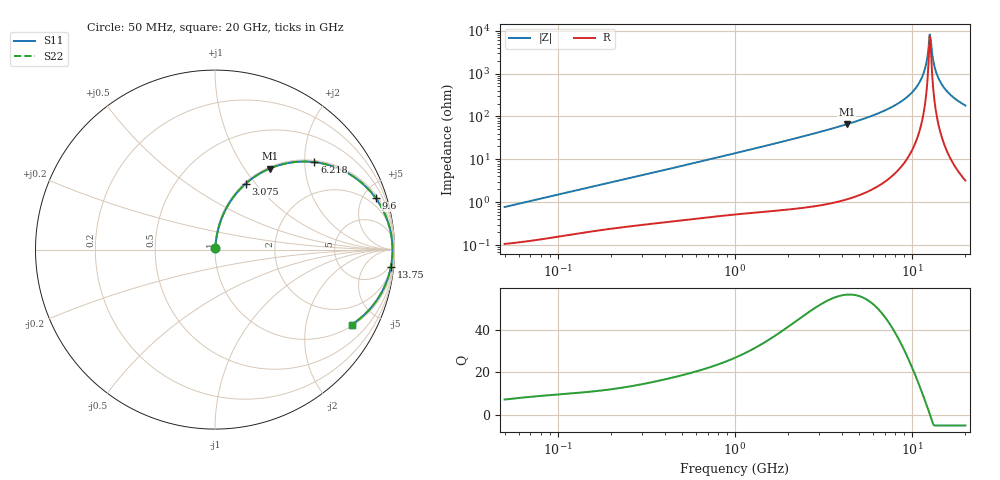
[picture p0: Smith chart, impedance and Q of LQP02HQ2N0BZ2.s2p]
!Murata Part Number: LQP02HQ2N0BZ2
!These Parameters are Measured in Series Mode Connection
!  o--[Z]--o
!Port1  Port2
!  o-------o
!Freq. Start=50[MHz] Stop=20[GHz], 401[Steps]
# Hz S RI R 50
!Freq.(Hz) S11(Real) S11(Imag) S21(Real) S21(Imag) S12(Real) S12(Imag) S22(Real) S22(Imag)
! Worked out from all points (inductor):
!   401 points, 50 MHz to 20 GHz, reference 50 ohm
!   read as one part in series: L = 2.43 nH near 51.52 MHz
!   highest Q = 56.4 at 4.276 GHz (marker M1), where L = 2.45 nH
!   self-resonance near 12.57 GHz
!   S11 on the Smith chart (normalised r, x): 50 MHz: 1.00, +0.02; 3.075 GHz: 1.02, +0.89; 6.218 GHz: 1.04, +2.23; 9.6 GHz: 1.24, +6.18; 13.75 GHz: 3, -20; 20 GHz: 1.06, -3.60
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5e7  0.00112 0.00765  0.9989 -0.00765  0.9989 -0.00765  0.00112 0.00765
1.364002e8  0.00232 0.0201  0.9977 -0.0201  0.9977 -0.0201  0.00232 0.0201
3.721004e8  0.00601 0.0521  0.994 -0.0521  0.994 -0.0521  0.00601 0.0521
1e9  0.0237 0.1347  0.9763 -0.1347  0.9763 -0.1347  0.0237 0.1347
2.728004e9  0.1371 0.334  0.8629 -0.334  0.8629 -0.334  0.1371 0.334
3.075291e9  0.1703 0.3664  0.8297 -0.3664  0.8297 -0.3664  0.1703 0.3664
4.275624e9  0.305 0.4516  0.695 -0.4516  0.695 -0.4516  0.305 0.4516
6.217679e9  0.5539 0.4874  0.4461 -0.4874  0.4461 -0.4874  0.5539 0.4874
7.442007e9  0.7021 0.4458  0.2979 -0.4458  0.2979 -0.4458  0.7021 0.4458
9.600142e9  0.8963 0.286  0.1037 -0.286  0.1037 -0.286  0.8963 0.286
1.050288e10  0.9452 0.2014  0.0548 -0.2014  0.0548 -0.2014  0.9452 0.2014
1.131968e10  0.9731 0.1226  0.0269 -0.1226  0.0269 -0.1226  0.9731 0.1226
1.183995e10  0.9833 0.0729  0.0167 -0.0729  0.0167 -0.0729  0.9833 0.0729
1.238412e10  0.9884 0.0221  0.0116 -0.0221  0.0116 -0.0221  0.9884 0.0221
1.257102e10  0.989 0.00504  0.011 -0.00504  0.011 -0.00504  0.989 0.00504
1.276073e10  0.9889 -0.012  0.0111 0.012  0.0111 0.012  0.9889 -0.012
1.295331e10  0.9883 -0.0291  0.0117 0.0291  0.0117 0.0291  0.9883 -0.0291
1.334722e10  0.9852 -0.063  0.0148 0.063  0.0148 0.063  0.9852 -0.063
1.375312e10  0.9798 -0.0966  0.0202 0.0966  0.0202 0.0966  0.9798 -0.0966
1.460232e10  0.9623 -0.1618  0.0377 0.1618  0.0377 0.1618  0.9623 -0.1618
1.573793e10  0.9289 -0.2377  0.0711 0.2377  0.0711 0.2377  0.9289 -0.2377
2e10  0.7607 -0.4179  0.2393 0.4179  0.2393 0.4179  0.7607 -0.4179
